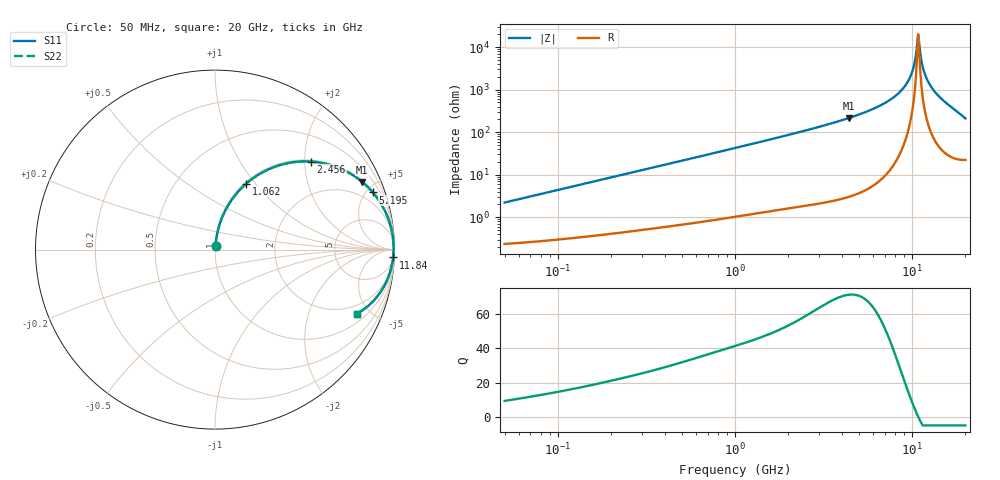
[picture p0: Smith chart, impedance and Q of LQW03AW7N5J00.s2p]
!Murata Part Number: LQW03AW7N5J00
!These Parameters are Measured in Series Mode Connection
!  o--[Z]--o
!Port1  Port2
!  o-------o
!Freq. Start=50[MHz] Stop=20[GHz], 401[Steps]
# Hz S RI R 50
!Freq.(Hz) S11(Real) S11(Imag) S21(Real) S21(Imag) S12(Real) S12(Imag) S22(Real) S22(Imag)
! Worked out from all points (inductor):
!   401 points, 50 MHz to 20 GHz, reference 50 ohm
!   read as one part in series: L = 7.01 nH near 51.52 MHz
!   highest Q = 71.3 at 4.406 GHz (marker M1), where L = 7.8 nH
!   self-resonance near 10.82 GHz
!   S11 on the Smith chart (normalised r, x): 50 MHz: 1.00, +0.04; 1.062 GHz: 1.02, +0.90; 2.456 GHz: 1.04, +2.15; 5.195 GHz: 1.08, +5.49; 11.84 GHz: 7, -45; 20 GHz: 1.45, -4.19
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5e7  0.00284 0.022  0.9972 -0.022  0.9972 -0.022  0.00284 0.022
1.364002e8  0.00686 0.0586  0.9931 -0.0586  0.9931 -0.0586  0.00686 0.0586
3.721004e8  0.0299 0.1533  0.9701 -0.1533  0.9701 -0.1533  0.0299 0.1533
1e9  0.1584 0.3532  0.8416 -0.3532  0.8416 -0.3532  0.1584 0.3532
1.061746e9  0.1744 0.3678  0.8256 -0.3678  0.8256 -0.3678  0.1744 0.3678
2.456456e9  0.5349 0.4903  0.4651 -0.4903  0.4651 -0.4903  0.5349 0.4903
2.728004e9  0.5908 0.4836  0.4092 -0.4836  0.4092 -0.4836  0.5908 0.4836
4.405649e9  0.8201 0.3772  0.1799 -0.3772  0.1799 -0.3772  0.8201 0.3772
5.194772e9  0.8793 0.3187  0.1207 -0.3187  0.1207 -0.3187  0.8793 0.3187
7.442007e9  0.9657 0.1714  0.0343 -0.1714  0.0343 -0.1714  0.9657 0.1714
8.516016e9  0.9833 0.1118  0.0167 -0.1118  0.0167 -0.1118  0.9833 0.1118
9.457416e9  0.9916 0.0641  0.00837 -0.0641  0.00837 -0.0641  0.9916 0.0641
1.004137e10  0.9942 0.0362  0.00582 -0.0362  0.00582 -0.0362  0.9942 0.0362
1.050288e10  0.995 0.015  0.005 -0.015  0.005 -0.015  0.995 0.015
1.066139e10  0.9951 0.00781  0.00494 -0.00781  0.00494 -0.00781  0.9951 0.00781
1.082228e10  0.995 0.000614  0.00499 -0.000614  0.00499 -0.000614  0.995 0.000614
1.115139e10  0.9946 -0.0139  0.00544 0.0139  0.00544 0.0139  0.9946 -0.0139
1.149051e10  0.9936 -0.0286  0.00636 0.0286  0.00636 0.0286  0.9936 -0.0286
1.183995e10  0.9922 -0.0435  0.00778 0.0435  0.00778 0.0435  0.9922 -0.0435
1.257102e10  0.9878 -0.0739  0.0122 0.0739  0.0122 0.0739  0.9878 -0.0739
1.396067e10  0.9738 -0.1297  0.0262 0.1297  0.0262 0.1297  0.9738 -0.1297
2e10  0.792 -0.3562  0.208 0.3562  0.208 0.3562  0.792 -0.3562
